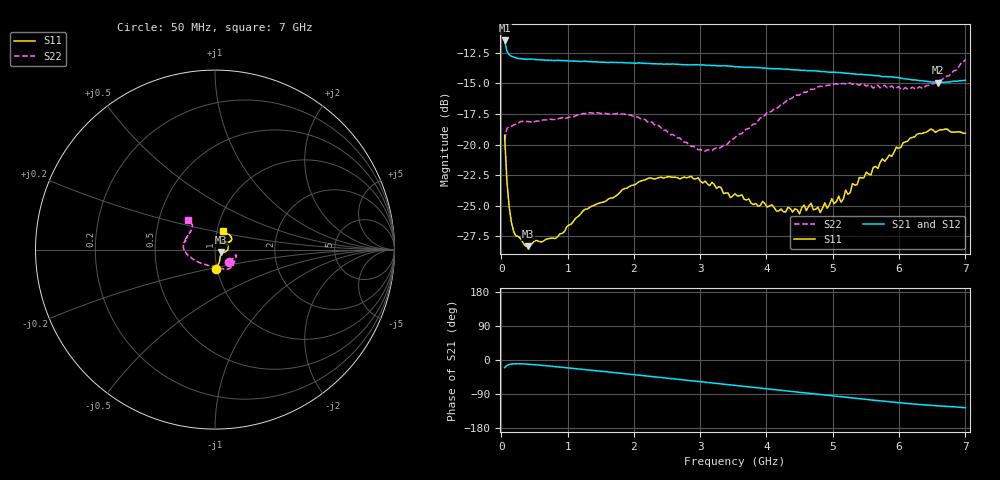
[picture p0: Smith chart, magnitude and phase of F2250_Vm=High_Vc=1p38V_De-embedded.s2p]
! Integrated Device Technology
! Corporate Headquarters
! 6024 Silver Creek Valley Road
! San Jose, CA 95138  USA
! Phone:  1-408-284-8200
! Toll Free:  1-800-223-1366
! Webpage:  http://www.idt.com/
! Timing and RF Division
! 515 Groton Road, Suite 102
! Westford, MA 01886-6024
! Device:  F2250
! Description: Voltage Variable RF Attenuator
! Frequency:  50.0 -  6000.00 MHz
! Package:  3x3 mm Thin QFN Plastic Package: 16 pin
! Ports:  2 RF, 3 DC
!  Pin  1  = GND
!  Pin  2  = NC
!  Pin  3  = RF1  = Port 1
!  Pin  4  = NC
!  Pin  5  = GND
!  Pin  6  = GND
!  Pin  7  = GND
!  Pin  8  = GND
!  Pin  9  = NC
!  Pin 10  = RF2  = Port 2
!  Pin 11  = NC
!  Pin 12  = GND
!  Pin 13  = GND
!  Pin 14  = VCNTRL
!  Pin 15  = VDD
!  Pin 16  = VMODE
! Vcntrl:  1.380 Volts
! Vmode:  +3.300 Volts
! Vdd:  +3.30  Volts
! Current:  1.331 mA
! Data:  The device was measured on a the F2250 evaluation board which has
!  individual transmission lines to the RF pins.  Data was collected
!  using a calibrated network analyzer.  The evaluation board was
!  de-embedded using a TRL calibration technique.
!  The reference plane is the edge of the package pin.
! Misc:  SN 10
!  Action Tracker AT0258
! Date Measured:  2014-11-26
! Date:  2015-10-15  MJV
! Note:
!  Integrated Device Technology supplies this data as a sample of measured
!  data at the package pin for this product.  Your particular data for this
!  product may vary.
!  Data was taken at 25 degrees C.
!  Integrated Device Technology reserves the right to change this data at anytime.
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# GHz S dB R 50
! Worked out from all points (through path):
!   201 points, 50 MHz to 7 GHz, reference 50 ohm
!   highest |S21| = -11.48 dB at 50 MHz (marker M1); lowest = -14.9 dB at 6.583 GHz (marker M2)
!   group delay of S21, straight-line fit = 49.9 ps
!   lowest |S11| = -28.3 dB at 397.5 MHz (marker M3), VSWR 1.08, Z = 53.6 - j1.72 ohm
!   |S11| at or under -10 dB: start of sweep to end of sweep
!   |S22| runs from -20.5 to -13.0 dB; largest |S21 - S12| = 0.00097
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0.05  -19.24 -86.5  -11.48 -20.0  -11.49 -20.0  -19.61 -40.5
0.08475  -23.00 -69.1  -12.36 -14.5  -12.37 -14.5  -18.68 -21.8
0.15425  -26.42 -51.9  -12.77 -10.6  -12.78 -10.6  -18.51 -14.6
0.22375  -27.50 -39.0  -12.91 -9.8  -12.92 -9.8  -18.31 -14.5
0.3975  -28.32 -24.7  -13.02 -11.0  -13.01 -11.0  -18.11 -16.1
0.8145  -27.70 -16.6  -13.12 -17.4  -13.10 -17.5  -17.95 -29.2
1.2315  -25.43 -15.9  -13.20 -24.8  -13.18 -24.8  -17.46 -40.5
2.37825  -22.70 6.0  -13.40 -45.6  -13.40 -45.6  -18.44 -65.8
3.07325  -22.99 26.2  -13.50 -58.7  -13.51 -58.7  -20.54 -101.7
3.525  -24.02 42.5  -13.63 -67.1  -13.63 -67.2  -19.44 -132.7
4.1505  -25.44 61.2  -13.81 -78.8  -13.78 -78.9  -17.06 -161.5
4.498  -25.67 59.3  -13.91 -85.4  -13.91 -85.4  -15.96 -172.1
4.67175  -24.81 59.0  -13.95 -88.7  -13.96 -88.7  -15.47 -175.8
4.7065  -25.34 59.6  -13.97 -89.3  -13.95 -89.4  -15.48 -176.3
4.81075  -25.57 55.4  -14.02 -91.2  -14.00 -91.3  -15.23 -178.2
5.08875  -24.22 46.3  -14.10 -96.5  -14.11 -96.5  -15.09 175.2
5.1235  -24.71 46.4  -14.12 -97.1  -14.12 -97.1  -15.02 174.3
5.193  -23.73 41.7  -14.16 -98.3  -14.15 -98.4  -15.04 173.0
5.85325  -20.85 28.8  -14.46 -110.2  -14.48 -110.3  -15.33 156.0
6.27025  -19.15 31.7  -14.73 -117.1  -14.71 -117.2  -15.42 142.9
6.583  -18.88 40.4  -14.93 -121.0  -14.91 -121.1  -14.83 134.2
7  -19.08 66.3  -14.73 -126.0  -14.72 -126.2  -13.05 132.9
